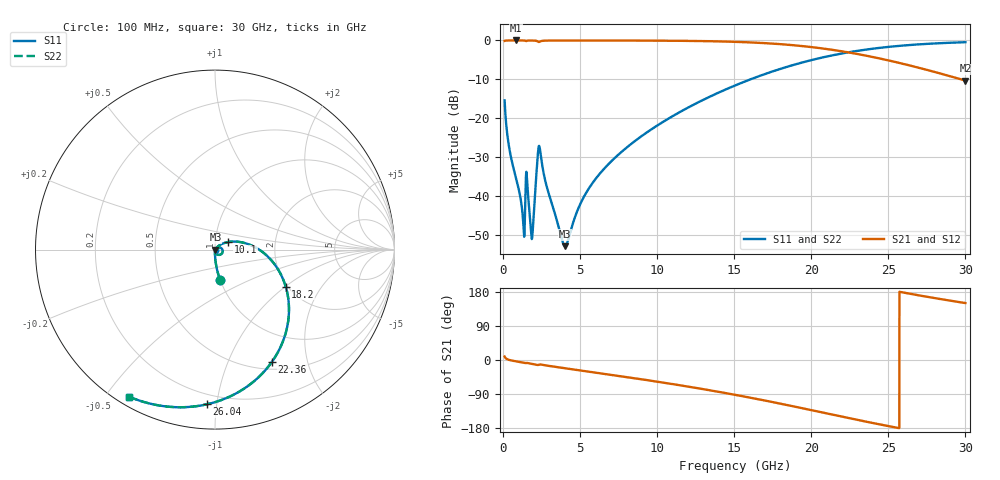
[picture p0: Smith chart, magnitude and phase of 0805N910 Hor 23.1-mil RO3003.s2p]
# GHz S MA R 50
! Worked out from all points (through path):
!   3201 points, 100 MHz to 30 GHz, reference 50 ohm
!   highest |S21| = -0.01 dB at 819.5 MHz (marker M1); lowest = -10.3 dB at 30 GHz (marker M2)
!   group delay of S21, straight-line fit = 20.2 ps
!   lowest |S11| = -52.7 dB at 4.024 GHz (marker M3), VSWR 1.00, Z = 50.2 - j0.0764 ohm
!   |S11| at or under -10 dB: start of sweep to 16.04 GHz
!   |S22| runs from -52.7 to -0.5 dB; largest |S21 - S12| = 0
!   S11 on the Smith chart (normalised r, x): 100 MHz: 1.00, -0.35; 10.1 GHz: 1.15, +0.10; 18.2 GHz: 1.96, -1.01; 22.36 GHz: 0.59, -1.46; 26.04 GHz: 0.14, -0.94; 30 GHz: 0.03, -0.58
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0.1  0.1704 -80.6  0.9851 9.3  0.9851 9.3  0.1704 -80.6
0.4083438  0.04093 -89.2  0.9987 0.1  0.9987 0.1  0.04093 -89.2
0.8194687  0.01779 -91.3  0.9992 -3.4  0.9992 -3.4  0.01779 -91.3
1.286656  0.005284 -80.8  0.9985 -6.7  0.9985 -6.7  0.005284 -80.8
1.595  0.01235 -71.8  0.9944 -8.0  0.9944 -8.0  0.01235 -71.8
1.865969  0.002844 -20.2  0.9971 -10.1  0.9971 -10.1  0.002844 -20.2
1.978094  0.005486 32.7  0.996 -11.0  0.996 -11.0  0.005486 32.7
2.239719  0.03179 19.7  0.9731 -13.2  0.9731 -13.2  0.03179 19.7
2.389219  0.04097 -43.1  0.9647 -11.8  0.9647 -11.8  0.04097 -43.1
2.875094  0.0125 -84.5  0.9955 -14.9  0.9955 -14.9  0.0125 -84.5
4.024375  0.002307 -19.2  0.9975 -21.8  0.9975 -21.8  0.002307 -19.2
5.089563  0.008635 47.1  0.9975 -27.9  0.9975 -27.9  0.008635 47.1
6.948969  0.02731 46.2  0.9969 -38.7  0.9969 -38.7  0.02731 46.2
10.06978  0.08273 30.3  0.9932 -57.6  0.9932 -57.6  0.08273 30.3
10.09781  0.0834 30.1  0.9931 -57.8  0.9931 -57.8  0.0834 30.1
15.05  0.2645 -2.8  0.9594 -91.8  0.9594 -91.8  0.2645 -2.8
18.19884  0.4446 -27.6  0.8896 -116.9  0.8896 -116.9  0.4446 -27.6
20.03956  0.5618 -43.2  0.8205 -132.6  0.8205 -132.6  0.5618 -43.2
22.35681  0.7012 -63.1  0.7054 -152.6  0.7054 -152.6  0.7012 -63.1
25.01978  0.8269 -85.1  0.554 -174.6  0.554 -174.6  0.8269 -85.1
26.03825  0.8628 -92.9  0.4968 177.6  0.4968 177.6  0.8628 -92.9
30  0.9488 -120.1  0.3057 150.3  0.3057 150.3  0.9488 -120.1
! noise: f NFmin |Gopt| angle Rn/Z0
0.1  0.0004134  0.8549  0.6667  0.0006082
3.417  0.007221  0.7361  18.52  0.005331
6.743  0.009693  0.6404  35.91  0.00463
10.06  0.01319  0.6206  52.27  0.005297
13.39  0.01716  0.6228  67.55  0.006013
16.7  0.02188  0.639  81.69  0.006784
20.03  0.0279  0.6665  95  0.007676
23.35  0.03593  0.7039  107.7  0.008752
26.67  0.04737  0.7499  120.2  0.01006
30  0.06469  0.8014  132.9  0.01148
